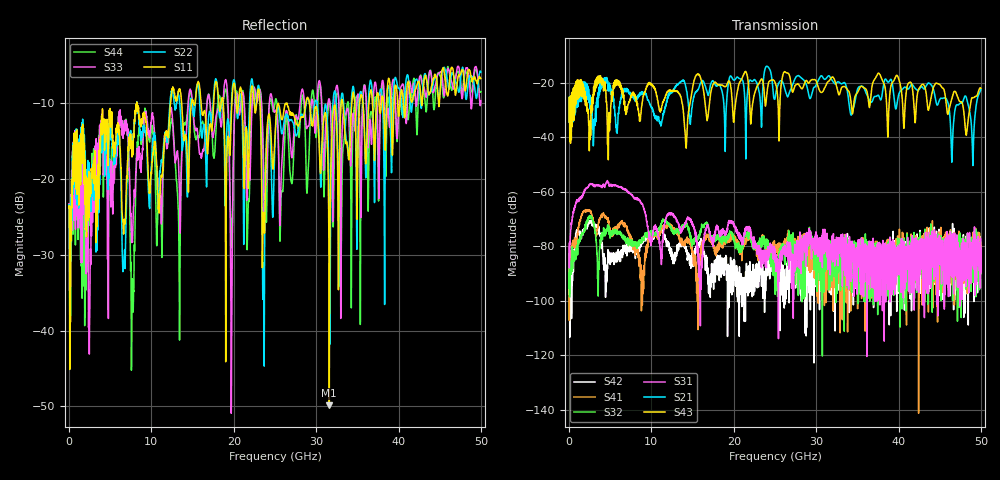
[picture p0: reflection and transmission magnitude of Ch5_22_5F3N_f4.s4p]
!Agilent Technologies,N5247A,US51170199,A.09.90.13
!Agilent N5247A: A.09.90.13
!Date: Wednesday, December 09, 2015 09:52:28
!Correction: S11(Full 4 Port(1,2,3,4))
!S12(Full 4 Port(1,2,3,4))
!S13(Full 4 Port(1,2,3,4))
!S14(Full 4 Port(1,2,3,4))
!S21(Full 4 Port(1,2,3,4))
!S22(Full 4 Port(1,2,3,4))
!S23(Full 4 Port(1,2,3,4))
!S24(Full 4 Port(1,2,3,4))
!S31(Full 4 Port(1,2,3,4))
!S32(Full 4 Port(1,2,3,4))
!S33(Full 4 Port(1,2,3,4))
!S34(Full 4 Port(1,2,3,4))
!S41(Full 4 Port(1,2,3,4))
!S42(Full 4 Port(1,2,3,4))
!S43(Full 4 Port(1,2,3,4))
!S44(Full 4 Port(1,2,3,4))
!S4P File: Measurements: <S11,S12,S13,S14>,
!<S21,S22,S23,S24>,
!<S31,S32,S33,S34>,
!<S41,S42,S43,S44>:
# Hz S  dB  R 50
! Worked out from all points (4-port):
!   3201 points, 10 MHz to 50 GHz, reference 50 ohm
!   strongest paths, dB at 10 MHz, 12.51 GHz, 25 GHz, 37.5 GHz, 50 GHz:
!     S43: -34.4, -23.2, -19.8, -16.6, -22.0
!     S21: -34.5, -23.5, -25.9, -24.6, -22.5
!     S31: -79.0, -68.3, -81.1, -78.8, -80.9
!     S32: -88.2, -74.7, -90.0, -85.6, -81.0
!     S41: -80.3, -73.8, -81.0, -93.1, -88.2
!     S42: -82.7, -84.9, -88.0, -90.3, -81.6
!   lowest |S11| = -49.9 dB at 31.6 GHz (marker M1), VSWR 1.01, Z = 49.9 + j0.303 ohm
!   |S11| at or under -10 dB: start of sweep to 8.216 GHz; 8.246 GHz to 12.34 GHz (4.09 GHz wide, 39.7 % of centre); 29.18 GHz to 33.03 GHz (3.855 GHz wide, 12.4 % of centre)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
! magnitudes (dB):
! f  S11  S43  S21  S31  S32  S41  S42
! 10 MHz  -23.8  -34.4  -34.5  -79.0  -88.2  -80.3  -82.7
! 4.618 GHz  -12.1  -31.9  -19.4  -56.2  -73.8  -70.2  -87.4
! 11.13 GHz  -20.1  -29.7  -35.8  -83.6  -72.5  -75.2  -74.4
! 31.6 GHz  -49.9  -19.3  -17.5  -80.0  -83.9  -86.9  -84.4
! 43.78 GHz  -8.6  -28.2  -20.3  -77.9  -84.5  -73.2  -76.4
! 46.5 GHz  -5.2  -25.6  -47.0  -91.4  -80.2  -94.2  -86.2
! 50 GHz  -6.7  -22.0  -22.5  -80.9  -81.0  -88.2  -81.6
